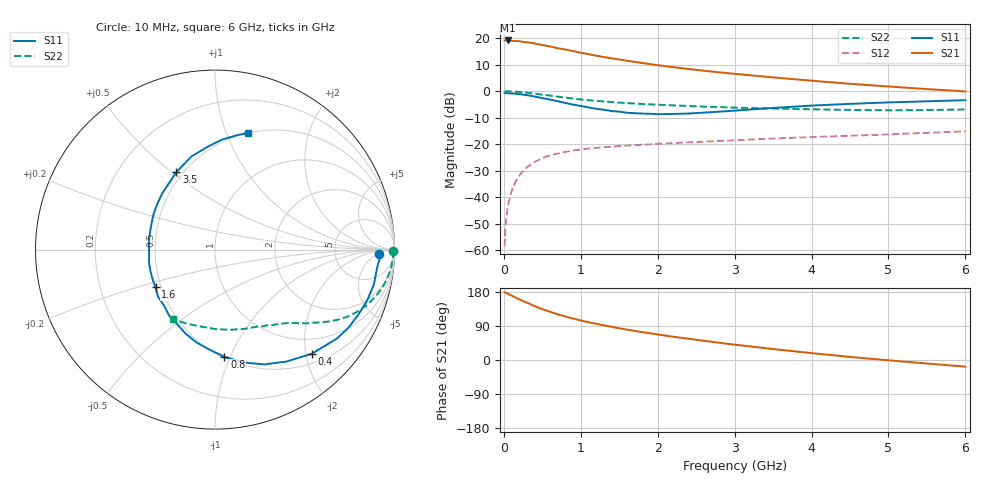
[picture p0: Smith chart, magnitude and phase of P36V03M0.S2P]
! SIEMENS Small Signal Semiconductors
! BFP181
! Si NPN RF Bipolar Junction Transistor in SOT143
! VCE = 6 V  IC = 3 mA
! Common Emitter S-Parameters:  March  1996
# GHz  S  MA  R  50
!  f  S11  S21  S12  S22
! GHz  MAG  ANG  MAG  ANG  MAG  ANG  MAG  ANG
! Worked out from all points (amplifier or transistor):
!   36 points, 10 MHz to 6 GHz, reference 50 ohm
!   highest |S21| = 19.1 dB at 50 MHz (marker M1)
!   |S21| within 3 dB of that: start of sweep to 715.7 MHz
!   unconditionally stable (mu >= 1): 2.197 GHz to end of sweep
!   at 250 MHz: K = 0.15, MSG = 24.3 dB, |S12| = -30.1 dB
!   at 1.4 GHz: K = 0.74, MSG = 16.6 dB, |S12| = -20.9 dB
!   at 6 GHz: K = 1.10, MAG = 5.6 dB, |S12| = -15.1 dB
!   lowest NFmin = 1.40 dB at 450 MHz
!   S11 on the Smith chart (normalised r, x): 10 MHz: 21, -6; 400 MHz: 0.68, -2.12; 800 MHz: 0.51, -0.95; 1.6 GHz: 0.47, -0.23; 3.5 GHz: 0.46, +0.52; 6 GHz: 0.50, +1.19
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0.01  0.9141 -1.4  8.975 178.8  0.0012 92.6  0.9937 -0.5
0.02  0.922 -2.5  9.022 178.2  0.0028 90.0  0.996 -1.1
0.05  0.9094 -6.0  9.029 174.8  0.0066 86.5  0.9911 -2.8
0.1  0.9062 -12.3  8.82 170.1  0.013 80.8  0.9871 -5.6
0.2  0.8773 -24.4  8.742 160.2  0.0254 75.8  0.9665 -11.0
0.3  0.8414 -36.0  8.343 151.5  0.0367 69.4  0.9356 -15.8
0.4  0.7927 -47.0  7.954 142.1  0.0464 63.6  0.9001 -20.2
0.5  0.7403 -57.4  7.399 134.2  0.0545 58.2  0.8601 -24.0
0.6  0.6961 -66.8  6.959 127.3  0.062 54.0  0.8243 -27.1
0.7  0.6474 -76.1  6.449 120.7  0.0669 50.3  0.7882 -29.7
0.8  0.5992 -85.0  6.094 114.6  0.0719 46.9  0.7561 -31.9
1  0.5272 -101.4  5.287 104.4  0.0794 42.1  0.6986 -35.6
1.1  0.4943 -109.7  4.991 99.6  0.0827 39.8  0.6757 -37.1
1.3  0.4475 -124.8  4.388 91.4  0.0877 36.6  0.6398 -39.9
1.6  0.3925 -147.6  3.747 80.2  0.0941 33.4  0.5976 -43.2
1.8  0.3785 -162.6  3.391 73.5  0.0979 32.0  0.5731 -45.6
2.2  0.3721 171.9  2.834 61.4  0.1052 29.4  0.5395 -50.4
2.8  0.4106 141.5  2.26 45.4  0.1156 26.4  0.5022 -58.5
3.5  0.4827 116.4  1.816 28.9  0.1279 23.5  0.4715 -69.4
4.5  0.576 93.8  1.377 8.1  0.1447 18.6  0.4437 -89.0
5.5  0.6436 80.1  1.095 -9.3  0.1643 14.9  0.4413 -110.1
6  0.6769 74.3  0.99 -17.5  0.1748 12.2  0.4525 -121.0
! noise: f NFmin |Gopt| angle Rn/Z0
0.45  1.4  0.56  17  0.36
0.9  1.5  0.45  35  0.34
1.8  1.85  0.25  82  0.36
